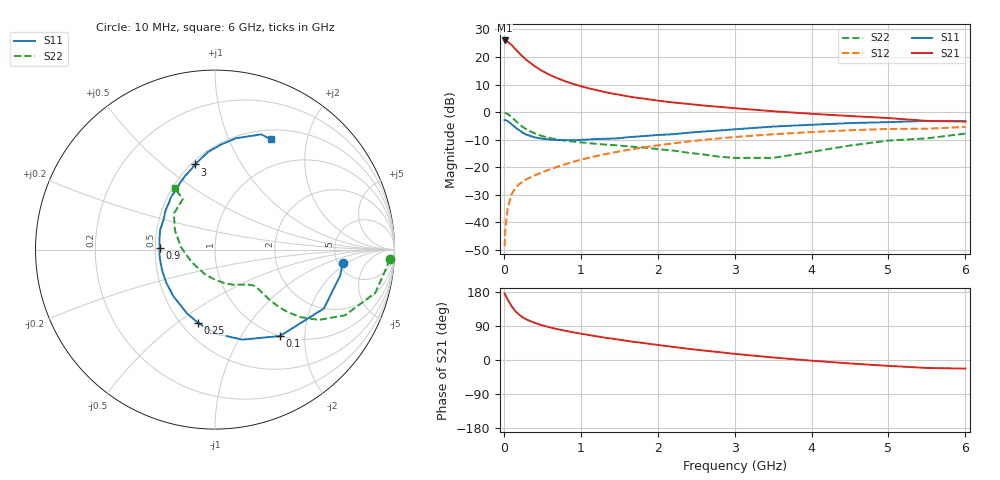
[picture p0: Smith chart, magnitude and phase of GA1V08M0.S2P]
! Infineon Technologies  Discrete & RF Semiconductors
! BF775
! Si NPN RF Bipolar Junction Transistor in SOT23
! VCE = 1 V  IC = 8 mA
! Common Emitter S-Parameters:  May  1996
# GHz  S  MA  R  50
!  f  S11  S21  S12  S22
! GHz  MAG  ANG  MAG  ANG  MAG  ANG  MAG  ANG
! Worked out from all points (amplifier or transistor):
!   36 points, 10 MHz to 6 GHz, reference 50 ohm
!   highest |S21| = 26.0 dB at 10 MHz (marker M1)
!   |S21| within 3 dB of that: start of sweep to 145 MHz
!   unconditionally stable (mu >= 1): 542.1 MHz to end of sweep
!   at 250 MHz: K = 0.66, MSG = 22.6 dB, |S12| = -25.2 dB
!   at 1.4 GHz: K = 1.17, MAG = 8.3 dB, |S12| = -14.8 dB
!   at 6 GHz: K = 1.03, MAG = -0.1 dB, |S12| = -5.4 dB
!   S11 on the Smith chart (normalised r, x): 10 MHz: 5.54, -1.68; 100 MHz: 1.00, -1.51; 250 MHz: 0.60, -0.60; 900 MHz: 0.53, +0.01; 3 GHz: 0.52, +0.65; 6 GHz: 0.62, +1.44
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0.01  0.717 -5.9  19.9 175.9  0.0037 87.5  0.9746 -3.1
0.02  0.7121 -11.8  19.62 171.3  0.0077 84.8  0.9601 -6.2
0.05  0.6896 -28.4  18.89 159.4  0.018 76.3  0.9248 -15.1
0.1  0.6024 -53.1  16.57 142.1  0.0321 66.3  0.8114 -26.8
0.15  0.5242 -73.1  13.84 128.8  0.0421 60.6  0.6986 -34.1
0.2  0.4689 -89.4  11.76 119.3  0.0494 57.5  0.6072 -38.3
0.25  0.4187 -103.1  10.02 111.9  0.0549 55.7  0.5328 -40.7
0.3  0.3877 -113.9  8.675 106.4  0.061 56.1  0.4812 -41.9
0.4  0.3482 -131.8  6.815 98.2  0.071 56.0  0.412 -42.6
0.5  0.3283 -145.8  5.56 91.4  0.081 57.1  0.3659 -42.5
0.6  0.3173 -157.2  4.714 86.1  0.0915 58.0  0.3375 -42.3
0.7  0.312 -166.1  4.098 81.2  0.1025 58.6  0.3181 -42.4
0.9  0.3079 178.5  3.242 73.1  0.1252 58.6  0.292 -43.2
1.1  0.3181 165.6  2.71 66.1  0.1478 58.2  0.2741 -45.8
1.3  0.3264 155.5  2.327 59.5  0.1705 56.8  0.259 -48.5
1.6  0.3487 142.9  1.941 50.5  0.2047 54.3  0.2397 -54.7
2.2  0.3968 123.1  1.493 34.6  0.2712 47.8  0.2005 -71.7
3  0.4871 103.2  1.177 16.2  0.3532 37.2  0.1476 -113.0
3.5  0.5461 94.0  1.036 6.6  0.396 30.2  0.1478 -151.7
4.5  0.6316 79.3  0.848 -9.1  0.4678 16.5  0.2475 154.4
5.5  0.692 68.1  0.691 -21.0  0.4998 2.8  0.3337 122.5
6  0.6881 63.2  0.674 -22.7  0.5368 -1.1  0.4076 123.3
